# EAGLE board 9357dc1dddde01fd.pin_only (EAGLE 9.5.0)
REV: B

Size 50.8 x 22.86 mm. Coordinates in mm from the lower left corner, seen from the top.
Outline: 2.54,0 48.26,0 arc90 50.8,2.54 50.8,20.32 arc90 48.26,22.86 2.54,22.86 arc90 0,20.32 0,2.54 arc90 2.54,0
Copper layers (1*16): Top 0.035mm / dielectric 1.5mm / Bottom 0.035mm
Design rules "adafruit *": minimum track width 8mil, minimum drill 15.5mil, track to track 7mil, track to pad 7mil, pad to pad 7mil, via to via 7mil, smd to smd 7mil, copper to edge 10mil, drill to drill 8mil, minimum pad ring 10mil, minimum via ring 8mil, stop-mask expansion 2mil, vias tented up to drill 20mil, thermal gap 10mil
Net classes: 1 power: width 0.305 mm; 2 gnd: width 0.254 mm
Holes 2.54 mm at 48.26,20.32 48.26,2.54

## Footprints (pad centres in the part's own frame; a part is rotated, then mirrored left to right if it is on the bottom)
0603-NO = smd 1.075 x 1: 1 -0.85,0; 2 0.85,0
RESPACK_4X0603 = smd 0.45 x 0.9: 1 -1.3,-0.85; 2 -0.4,-0.85; 3 0.4,-0.85; 4 1.3,-0.85; 5 1.3,0.85; 6 0.4,0.85; 7 -0.4,0.85; 8 -1.3,0.85
0805-NO = smd 1.24 x 1.5: 1 -0.95,0; 2 0.95,0
CHIPLED_0805_NOOUTLINE = smd 1.2 x 1.2: A 0,-1.05; C 0,1.05
JST_SH4 = smd 0.6 x 1.55: 1 -1.5,2.514; 2 -0.5,2.514; 3 0.5,2.514; 4 1.5,2.514 | smd 1.2 x 1.8: MT1 -2.8,-1.386; MT2 2.8,-1.386
SOD-123 = smd 1.4 x 1.4: A 1.85,0; C -1.85,0
B1,27 = smd 1.27 x 1.27: TP 0,0
1X16_ROUND = drill 1 pad 1.676: 1 -19.05,0; 2 -16.51,0; 3 -13.97,0; 4 -11.43,0; 5 -8.89,0; 6 -6.35,0; 7 -3.81,0; 8 -1.27,0; 9 1.27,0; 10 3.81,0; 11 6.35,0; 12 8.89,0; 13 11.43,0; 14 13.97,0; 15 16.51,0; 16 19.05,0
1X12_ROUND = drill 1 pad 1.676: 1 -13.97,0; 2 -11.43,0; 3 -8.89,0; 4 -6.35,0; 5 -3.81,0; 6 -1.27,0; 7 1.27,0; 8 3.81,0; 9 6.35,0; 10 8.89,0; 11 11.43,0; 12 13.97,0
LED3535 = smd 1 x 0.85: 1 -1.75,0.875; 2 -1.75,-0.875; 3 1.75,-0.875; 4 1.75,0.875
SOT23-R = smd 0.635 x 1.016: 1 -0.95,-1; 2 0.95,-1; 3 0,1
RESPACK_4X0603_NO = smd 0.45 x 0.9: 1 -1.3,-0.85; 2 -0.4,-0.85; 3 0.4,-0.85; 4 1.3,-0.85; 5 1.3,0.85; 6 0.4,0.85; 7 -0.4,0.85; 8 -1.3,0.85
BTN_KMR2_4.6X2.8 = smd 0.9 x 0.9: A 2.05,0.8; A' -2.05,0.8; B 2.05,-0.8; B' -2.05,-0.8
TESTPOINT_ROUND_1.5MM = smd 1.5 x 1.5: P$1 0,0
SOIC8_150MIL = smd 0.6 x 2.2: 1 -1.905,-2.6; 2 -0.635,-2.6; 3 0.635,-2.6; 4 1.905,-2.6; 5 1.905,2.6; 6 0.635,2.6; 7 -0.635,2.6; 8 -1.905,2.6
SOT23-5 = smd 0.55 x 1.2: 1 -0.95,-1.3; 2 0,-1.3; 3 0.95,-1.3; 4 0.95,1.3; 5 -0.95,1.3
TQFP64 = smd 1.143 x 0.305: 1 -5.7,3.75; 2 -5.7,3.25; 3 -5.7,2.75; 4 -5.7,2.25; 5 -5.7,1.75; 6 -5.7,1.25; 7 -5.7,0.75; 8 -5.7,0.25; 9 -5.7,-0.25; 10 -5.7,-0.75; 11 -5.7,-1.25; 12 -5.7,-1.75; 13 -5.7,-2.25; 14 -5.7,-2.75; 15 -5.7,-3.25; 16 -5.7,-3.75; 33 5.7,-3.75; 34 5.7,-3.25; 35 5.7,-2.75; 36 5.7,-2.25; 37 5.7,-1.75; 38 5.7,-1.25; 39 5.7,-0.75; 40 5.7,-0.25; 41 5.7,0.25; 42 5.7,0.75; 43 5.7,1.25; 44 5.7,1.75; 45 5.7,2.25; 46 5.7,2.75; 47 5.7,3.25; 48 5.7,3.75 | smd 0.305 x 1.143: 17 -3.75,-5.7; 18 -3.25,-5.7; 19 -2.75,-5.7; 20 -2.25,-5.7; 21 -1.75,-5.7; 22 -1.25,-5.7; 23 -0.75,-5.7; 24 -0.25,-5.7; 25 0.25,-5.7; 26 0.75,-5.7; 27 1.25,-5.7; 28 1.75,-5.7; 29 2.25,-5.7; 30 2.75,-5.7; 31 3.25,-5.7; 32 3.75,-5.7; 49 3.75,5.7; 50 3.25,5.7; 51 2.75,5.7; 52 2.25,5.7; 53 1.75,5.7; 54 1.25,5.7; 55 0.75,5.7; 56 0.25,5.7; 57 -0.25,5.7; 58 -0.75,5.7; 59 -1.25,5.7; 60 -1.75,5.7; 61 -2.25,5.7; 62 -2.75,5.7; 63 -3.25,5.7; 64 -3.75,5.7
FIDUCIAL_1MM = smd 1 x 1: 1 0,0
MOUNTINGHOLE_2.5_PLATED = drill 2.5 pad 3.2: P$1 0,0
JSTPH2 = smd 1 x 4.6: 1 -1,-3.7; 2 1,-3.7 | smd 1.6 x 3.4: NC1 -3.4,1.5; NC2 3.4,1.5
XTAL3215 = smd 1.1 x 1.9: P$1 1.2,0; P$2 -1.2,0
2X05_1.27MM_SMT = smd 0.65 x 2.6: 1 -2.54,-1.85; 2 -2.54,1.85; 3 -1.27,-1.85; 4 -1.27,1.85; 5 0,-1.85; 6 0,1.85; 7 1.27,-1.85; 8 1.27,1.85; 9 2.54,-1.85; 10 2.54,1.85
MICROSD = smd 0.7 x 1.5: 1 9,-10.64; 2 7.9,-10.24; 3 6.8,-10.64; 4 5.7,-11.04; 5 4.6,-10.64; 6 3.5,-11.04; 7 2.4,-10.64; 8 1.3,-10.64 | smd 1.8 x 1.4: CD1 2,-0.44; CD2 8,-0.44 | smd 1.4 x 1.9: MT1 0.4,-13.54; MT2 13.6,-14.44
USB_C_CUSB31-CFM2AX-01-X = smd 0.575 x 1.15: A1B12 -3.2,3.545; A4B9 -2.4,3.545; B1A12 3.2,3.545; B4A9 2.4,3.545 | smd 0.275 x 1.15: A5 -1.25,3.545; A6 -0.25,3.545; A7 0.25,3.545; A8 1.25,3.545; B5 1.75,3.545; B6 0.75,3.545; B7 -0.75,3.545; B8 -1.75,3.545 | drill 0.6 pad 1 long: M1 -4.32,2.97; M2 4.32,2.97; M3 -4.32,-1.21; M4 4.32,-1.21 | hole 0.65: 2.89,2.47; -2.89,2.47
CRYSTAL_2.5X2 = smd 0.9 x 0.75: 1 -0.825,-0.625; 2 0.825,-0.625; 3 0.825,0.625; 4 -0.825,0.625

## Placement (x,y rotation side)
C1  0.1uF  [0603-NO]  9.33,4.19 0 top
C2  22pF  [RESPACK_4X0603]  22.1,12.83 90 top
C3  10µF  [0805-NO]  16.19,16.45 270 top
C4  1uF  [0603-NO]  45.09,18.16 0 top
C5  10uF  [0805-NO]  24.45,17.73 90 top
C6  10µF  [0805-NO]  12.9,9.25 0 top
C7  1uF  [0603-NO]  26.18,17.53 90 top
C8  10µF  [0805-NO]  15.36,13.86 0 top
C9  10µF  [0805-NO]  39.88,5.78 0 top
C10  1uF  [0603-NO]  23.68,5.64 90 top
C11  1uF  [0603-NO]  14.34,6.41 270 top
C12  10µF  [0805-NO]  40.89,15.81 90 top
C13  10µF  [0805-NO]  21.21,6.73 180 top
C14  1uF  [0603-NO]  13.45,4.15 0 top
C15  0.1uF  [0603-NO]  26.23,7.43 270 top
C16  1uF  [0603-NO]  43.12,6.67 0 top
C17  1uF  [0603-NO]  25.97,4.57 180 top
CHG  ORANGE  [CHIPLED_0805_NOOUTLINE]  2.41,5.59 270 top
CONN1  STEMMA_I2C_QT  [JST_SH4]  48.01,8.38 90 top
D4  MBR054  [SOD-123]  11.37,12.19 180 top
D+  TPB1,27  [B1,27]  2.54,12.7 0 bottom
D-  TPB1,27  [B1,27]  2.54,10.16 0 bottom
FB2  ferrite  [0805-NO]  20.95,4.89 0 top
JP1  [1X16_ROUND]  25.4,1.27 180 top
JP3  [1X12_ROUND]  30.48,21.59 0 top
L  RED  [CHIPLED_0805_NOOUTLINE]  2.65,17.36 90 top
LED1  WS2812B3535  [LED3535]  16.93,5.73 270 top
Q3  DMG3405  [SOT23-R]  9.65,9.72 0 top
R1  10K  [RESPACK_4X0603_NO]  43.05,9.78 90 top
R2  1K  [0603-NO]  6.02,4.19 0 top
R3  10K  [0603-NO]  19.43,10.29 90 top
R4  100K  [0603-NO]  44.07,5.02 180 top
R5  5.1K  [0603-NO]  6.22,5.71 180 top
R6  5.1K  [0603-NO]  8,12.19 90 top
R7  2.2K  [0603-NO]  5.65,19.3 270 top
R8  5.1K  [0603-NO]  18.61,17.78 0 top
R9  100K  [RESPACK_4X0603_NO]  22.03,17.34 90 top
R10  100K  [0603-NO]  39.88,4.25 180 top
SW1  KMR2  [BTN_KMR2_4.6X2.8]  10.54,6.54 180 top
TP1  [TESTPOINT_ROUND_1.5MM]  32.26,9.27 0 bottom
TP2  [TESTPOINT_ROUND_1.5MM]  32.26,12 0 bottom
TP3  [TESTPOINT_ROUND_1.5MM]  25.15,14.99 0 bottom
U1  25Q16  [SOIC8_150MIL]  46.42,14.85 90 top
U2  AP2112-3.3  [SOT23-5]  17.02,10.67 0 top
U3  MCP73831T-2ACI/OT  [SOT23-5]  18.86,15.11 0 top
U$3  STM32F405R  [TQFP64]  33.4,11.18 0 top
U$5  FIDUCIAL_1MM  [FIDUCIAL_1MM]  5.33,18.92 0 bottom
U$13  [PCBFEAT-REV-040]  5.08,11.75 0 bottom
U$24  [FEATHER_STM32F405_TOP]  0,0 0 top
U$31  MOUNTINGHOLE2.5  [MOUNTINGHOLE_2.5_PLATED]  2.54,20.32 270 top
U$32  MOUNTINGHOLE2.5  [MOUNTINGHOLE_2.5_PLATED]  2.54,2.54 270 top
U$34  FIDUCIAL_1MM  [FIDUCIAL_1MM]  10.48,20.89 270 top
U$35  FIDUCIAL_1MM  [FIDUCIAL_1MM]  46.4,0.77 270 top
U$37  FIDUCIAL_1MM  [FIDUCIAL_1MM]  46.48,1.08 0 bottom
U$40  [FEATHER_STM32F405_BOT]  50.8,0 0 bottom
X1  JSTPH  [JSTPH2]  10.92,19.3 0 top
X2  32.768  [XTAL3215]  24.69,14.07 90 top
X3  [2X05_1.27MM_SMT]  11.43,8.26 90 bottom
X5  [MICROSD]  34.92,18.41 270 bottom
X6  [USB_C_CUSB31-CFM2AX-01-X]  2.67,11.56 270 top
Y1  12mhz  [CRYSTAL_2.5X2]  23.37,9.53 180 top

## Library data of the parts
C1-C7 C9-C17 CHG CONN1 D4 FB2 JP1 JP3 L LED1 Q3 R1-R10 SW1 TP1-TP3 U1-U3 X1 X3 X5 X6 Y1 = microbuilder
C8 = microbuilder; COMPANY: ADAFRUIT INDUSTRIES; DRAWN: KTOWN; REV: B
D+ D- = testpad
U$3 = adafruit_micro
U$5 U$31 U$32 U$34 U$35 U$37 = microbuilder; BOM: EXCLUDE
U$13 = microbuilder; REV: B
U$24 U$40 = feather_silks
X2 = adafruit2

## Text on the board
tPlace: I2C

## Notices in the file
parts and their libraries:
microbuilder: This work is placed in the public domain, and may be freely used for commercial and non-commercial work with the following conditions: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
